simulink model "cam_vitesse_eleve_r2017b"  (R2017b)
settings: Solver=VariableStepAuto  StartTime=0.0  StopTime=10.0  RelTol=1e-3
model workspace (MAT data in the model file):
  distance = 10
  w_s_exp = 90

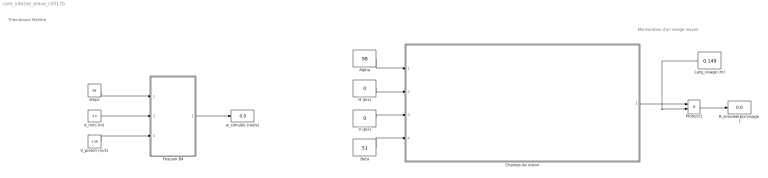
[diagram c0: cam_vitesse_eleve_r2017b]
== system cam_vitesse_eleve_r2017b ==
  note: Mensuration d'un visage moyen
  note: Thématique Matière
  Alpha : Constant  Value=98
  Beta : Constant  Value=51
  Champs de vision : Subsystem
  Foscam B4 : Subsystem
  H (pix) : Constant  Value=0
  Larg_visage (m) : Constant  Value=0.149
  Product1 : Product
  R_simulée(pix/visage) : Display
  V (pix) : Constant  Value=0
  V_pieton (m/s) : Constant  Value=1.38
  d_mini (m) : Constant  Value=3.5
  steps : Constant  Value=64
  w_simulée (rad/s) : Display
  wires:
  Product1/1 -> R_simulée(pix/visage)/1
  Larg_visage (m)/1 -> Product1/2
  Alpha/1 -> Champs de vision/1(alpha)
  H (pix)/1 -> Champs de vision/2(In2)
  V (pix)/1 -> Champs de vision/3(In3)
  Beta/1 -> Champs de vision/4(beta)
  Champs de vision/1(Out1) -> Product1/1
  steps/1 -> Foscam B4/1(In1)
  d_mini (m)/1 -> Foscam B4/2(In2)
  V_pieton (m/s)/1 -> Foscam B4/3(In3)
  Foscam B4/1(Out1) -> w_simulée (rad/s)/1

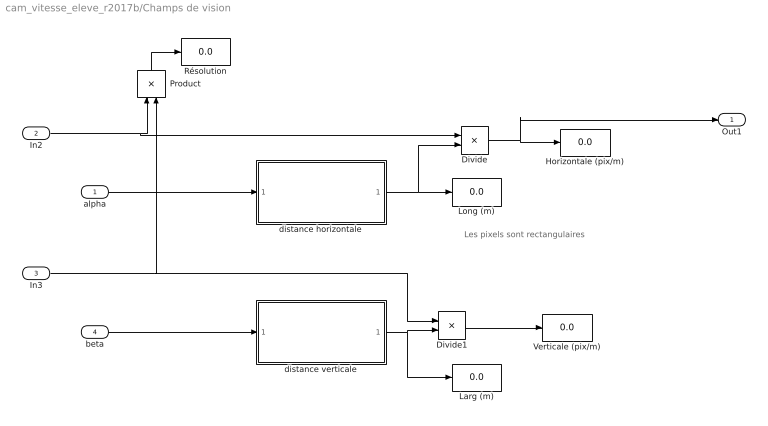
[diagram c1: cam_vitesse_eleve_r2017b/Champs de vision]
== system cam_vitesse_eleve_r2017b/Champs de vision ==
  note: Les pixels sont rectangulaires
  alpha : Inport
  In2 : Inport  Port=2
  In3 : Inport  Port=3
  beta : Inport  Port=4
  Divide : Product  Inputs=*/
  Divide1 : Product  Inputs=*/
  Horizontale (pix/m) : Display
  Larg (m) : Display
  Long (m) : Display
  Product : Product
  Résolution : Display
  Verticale (pix/m) : Display
  distance horizontale : MATLAB Function  TreatAsAtomicUnit=on
  distance verticale : MATLAB Function  TreatAsAtomicUnit=on
  Out1 : Outport  VectorParamsAs1DForOutWhenUnconnected=on
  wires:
  alpha/1 -> distance horizontale/1(alpha)
  distance verticale/1(Larg) -> Divide1/2, Larg (m)/1
  Product/1 -> Résolution/1
  distance horizontale/1(Long) -> Long (m)/1, Divide/2
  In2/1 -> Product/1, Divide/1
  Divide/1 -> Out1/1, Horizontale (pix/m)/1
  beta/1 -> distance verticale/1(beta)
  In3/1 -> Divide1/1, Product/2
  Divide1/1 -> Verticale (pix/m)/1

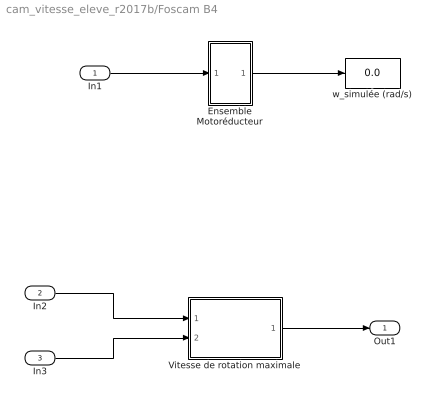
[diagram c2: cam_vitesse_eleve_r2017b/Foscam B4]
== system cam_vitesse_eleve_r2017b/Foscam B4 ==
  In1 : Inport
  In2 : Inport  Port=2
  In3 : Inport  Port=3
  Ensemble Motoréducteur : Subsystem
  Vitesse de rotation maximale : MATLAB Function  TreatAsAtomicUnit=on
  w_simulée (rad/s) : Display
  Out1 : Outport
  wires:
  Ensemble Motoréducteur/1(w_s) -> w_simulée (rad/s)/1
  In2/1 -> Vitesse de rotation maximale/1(d_mini)
  In1/1 -> Ensemble Motoréducteur/1(s)
  Vitesse de rotation maximale/1(w_max) -> Out1/1
  In3/1 -> Vitesse de rotation maximale/2(V_pieton)

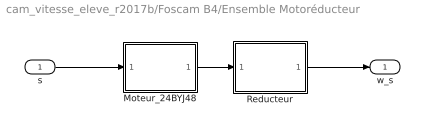
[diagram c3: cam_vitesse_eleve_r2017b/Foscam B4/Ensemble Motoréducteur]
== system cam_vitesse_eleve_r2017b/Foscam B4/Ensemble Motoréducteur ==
  s : Inport
  Moteur_24BYJ48 : MATLAB Function  TreatAsAtomicUnit=on
  Reducteur : MATLAB Function  TreatAsAtomicUnit=on
  w_s : Outport  VectorParamsAs1DForOutWhenUnconnected=on
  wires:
  Moteur_24BYJ48/1(w_m) -> Reducteur/1(w_e)
  s/1 -> Moteur_24BYJ48/1(s)
  Reducteur/1(w_s) -> w_s/1

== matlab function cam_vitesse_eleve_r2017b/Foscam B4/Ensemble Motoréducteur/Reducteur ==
function w_s = fcn(w_e)

r = 1/64; %rapport de transmission
w_s = (w_e*r);

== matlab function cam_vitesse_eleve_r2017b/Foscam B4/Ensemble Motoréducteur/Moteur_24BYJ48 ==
function w_m = fcn(s)

stepper = 360/s; %résultat en °/pas
w = 4.08; %tr/s
w_m = w*(2*pi); %résultat en rad/s

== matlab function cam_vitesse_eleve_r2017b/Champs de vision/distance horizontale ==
function Long = fcn(alpha)

distance  = 6;

Long = 2*distance*tan((alpha*(pi/180))/2);

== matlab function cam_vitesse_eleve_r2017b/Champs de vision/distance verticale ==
function Larg = fcn(beta)

distance  = 6;

Larg = 2*distance*tan(beta*(pi/180)/2);

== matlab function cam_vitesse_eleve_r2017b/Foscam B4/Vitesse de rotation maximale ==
function w_max = fcn(d_mini,V_pieton)

w_max = V_pieton/d_mini;
